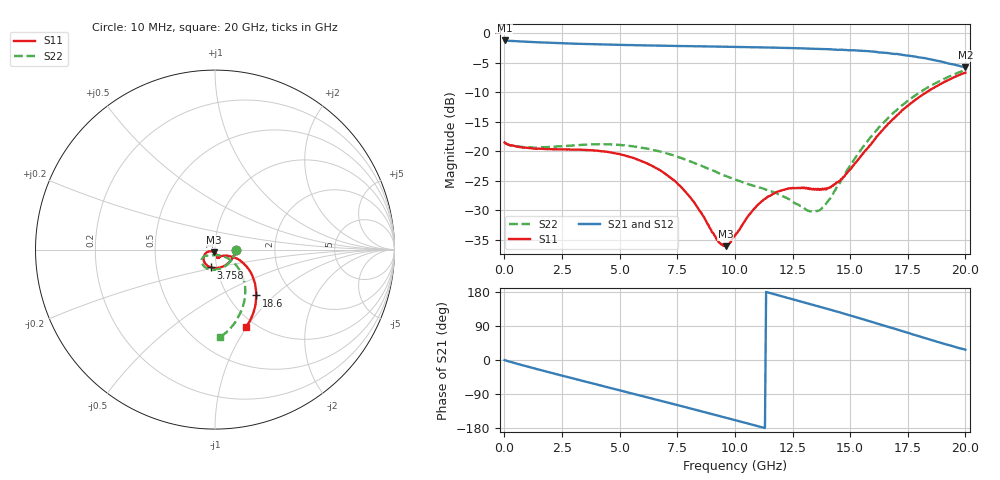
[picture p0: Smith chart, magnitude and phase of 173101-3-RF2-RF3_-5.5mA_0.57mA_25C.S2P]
!  2-Port S-parameters saved by WinCal
! VAR MeasName=S-Parameters (CALIBRATED_DATA) read from VNA (N5242A)
! VAR MeasDate=2017-7-20 9:27:09
! VAR NAME=173101-3-RF2-RF3_-5.5mA_0.57mA_25C
! VAR FILENAME=173101-3-RF2-RF3_-5.5mA_0.57mA_25C.S2P
! VAR DATE=2017-7-20 9:27:09
! VAR PHYS_PORTS=1,2
# Hz S DB R 50
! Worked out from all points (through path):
!   401 points, 10 MHz to 20 GHz, reference 50 ohm
!   highest |S21| = -1.19 dB at 10 MHz (marker M1); lowest = -5.8 dB at 20 GHz (marker M2)
!   group delay of S21, straight-line fit = 45.7 ps
!   lowest |S11| = -36.1 dB at 9.605 GHz (marker M3), VSWR 1.03, Z = 49.4 - j1.43 ohm
!   |S11| at or under -10 dB: start of sweep to 18.3 GHz
!   |S22| runs from -30.2 to -6.2 dB; largest |S21 - S12| = 0.0079
!   S11 on the Smith chart (normalised r, x): 10 MHz: 1.27, -0.00; 3.758 GHz: 0.94, -0.19; 18.6 GHz: 1.34, -0.78; 20 GHz: 0.90, -0.99
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1e7  -18.51 -0.7  -1.19 -0.3  -1.19 -0.3  -18.48 -0.8
1.559225e9  -19.55 -51.7  -1.51 -26.4  -1.52 -26.3  -19.31 -51.9
3.358325e9  -19.74 -94.6  -1.78 -54.5  -1.78 -54.5  -18.91 -92.3
3.758125e9  -19.81 -102.8  -1.82 -60.7  -1.82 -60.7  -18.84 -99.4
5.2074e9  -20.68 -128.9  -1.97 -83.2  -1.98 -83.1  -18.98 -121.4
6.70665e9  -23.09 -151.1  -2.07 -106.5  -2.06 -106.4  -19.97 -138.1
7.90605e9  -27.09 -162.1  -2.14 -125.1  -2.15 -125.0  -21.48 -146.2
8.555725e9  -30.53 -160.9  -2.18 -135.5  -2.18 -135.2  -22.45 -147.9
9.30535e9  -35.46 -133.7  -2.24 -147.4  -2.23 -147.3  -23.73 -146.7
9.6052e9  -36.10 -112.2  -2.26 -152.2  -2.25 -152.0  -24.19 -145.8
1.0005e10  -34.31 -87.7  -2.29 -158.6  -2.29 -158.5  -24.78 -143.3
1.085458e10  -29.65 -69.8  -2.34 -172.3  -2.35 -172.1  -25.90 -137.1
1.145428e10  -27.64 -69.9  -2.39 177.9  -2.39 178.1  -26.64 -131.9
1.24038e10  -26.26 -72.6  -2.48 162.1  -2.47 162.3  -28.25 -119.7
1.335332e10  -26.47 -66.4  -2.59 146.2  -2.58 146.3  -30.15 -90.6
1.38031e10  -26.34 -56.7  -2.67 138.4  -2.68 138.6  -29.52 -67.0
1.455272e10  -25.08 -37.4  -2.75 125.7  -2.75 125.8  -25.39 -40.6
1.575212e10  -19.49 -22.8  -3.01 103.9  -3.01 104.1  -18.29 -34.9
1.670165e10  -15.19 -25.6  -3.35 86.5  -3.40 86.5  -14.15 -41.8
1.76012e10  -11.96 -34.9  -3.80 70.1  -3.79 70.3  -11.14 -52.6
1.86007e10  -9.28 -48.0  -4.50 51.3  -4.53 51.7  -8.65 -66.4
2e10  -6.66 -68.2  -5.75 27.1  -5.79 27.8  -6.22 -86.7
